PROGRAM MAIN
VAR
Err_Ack AT %Q* :BOOL;
Run AT %Q* :BOOL:=TRUE;
Restart AT %Q* :BOOL;
Com_err AT %I* :BOOL;
FB_err AT %I*:BOOL;
	input1 AT %I*: BOOL;
END_VAR

Err_Ack:=input1;//链接到一个按钮，方便复位。用了4个OR功能块，实现四个输入，独立控制4个输出。用于检测EL6900+EL1904+EL2904的功能性测试。

END_PROGRAM
